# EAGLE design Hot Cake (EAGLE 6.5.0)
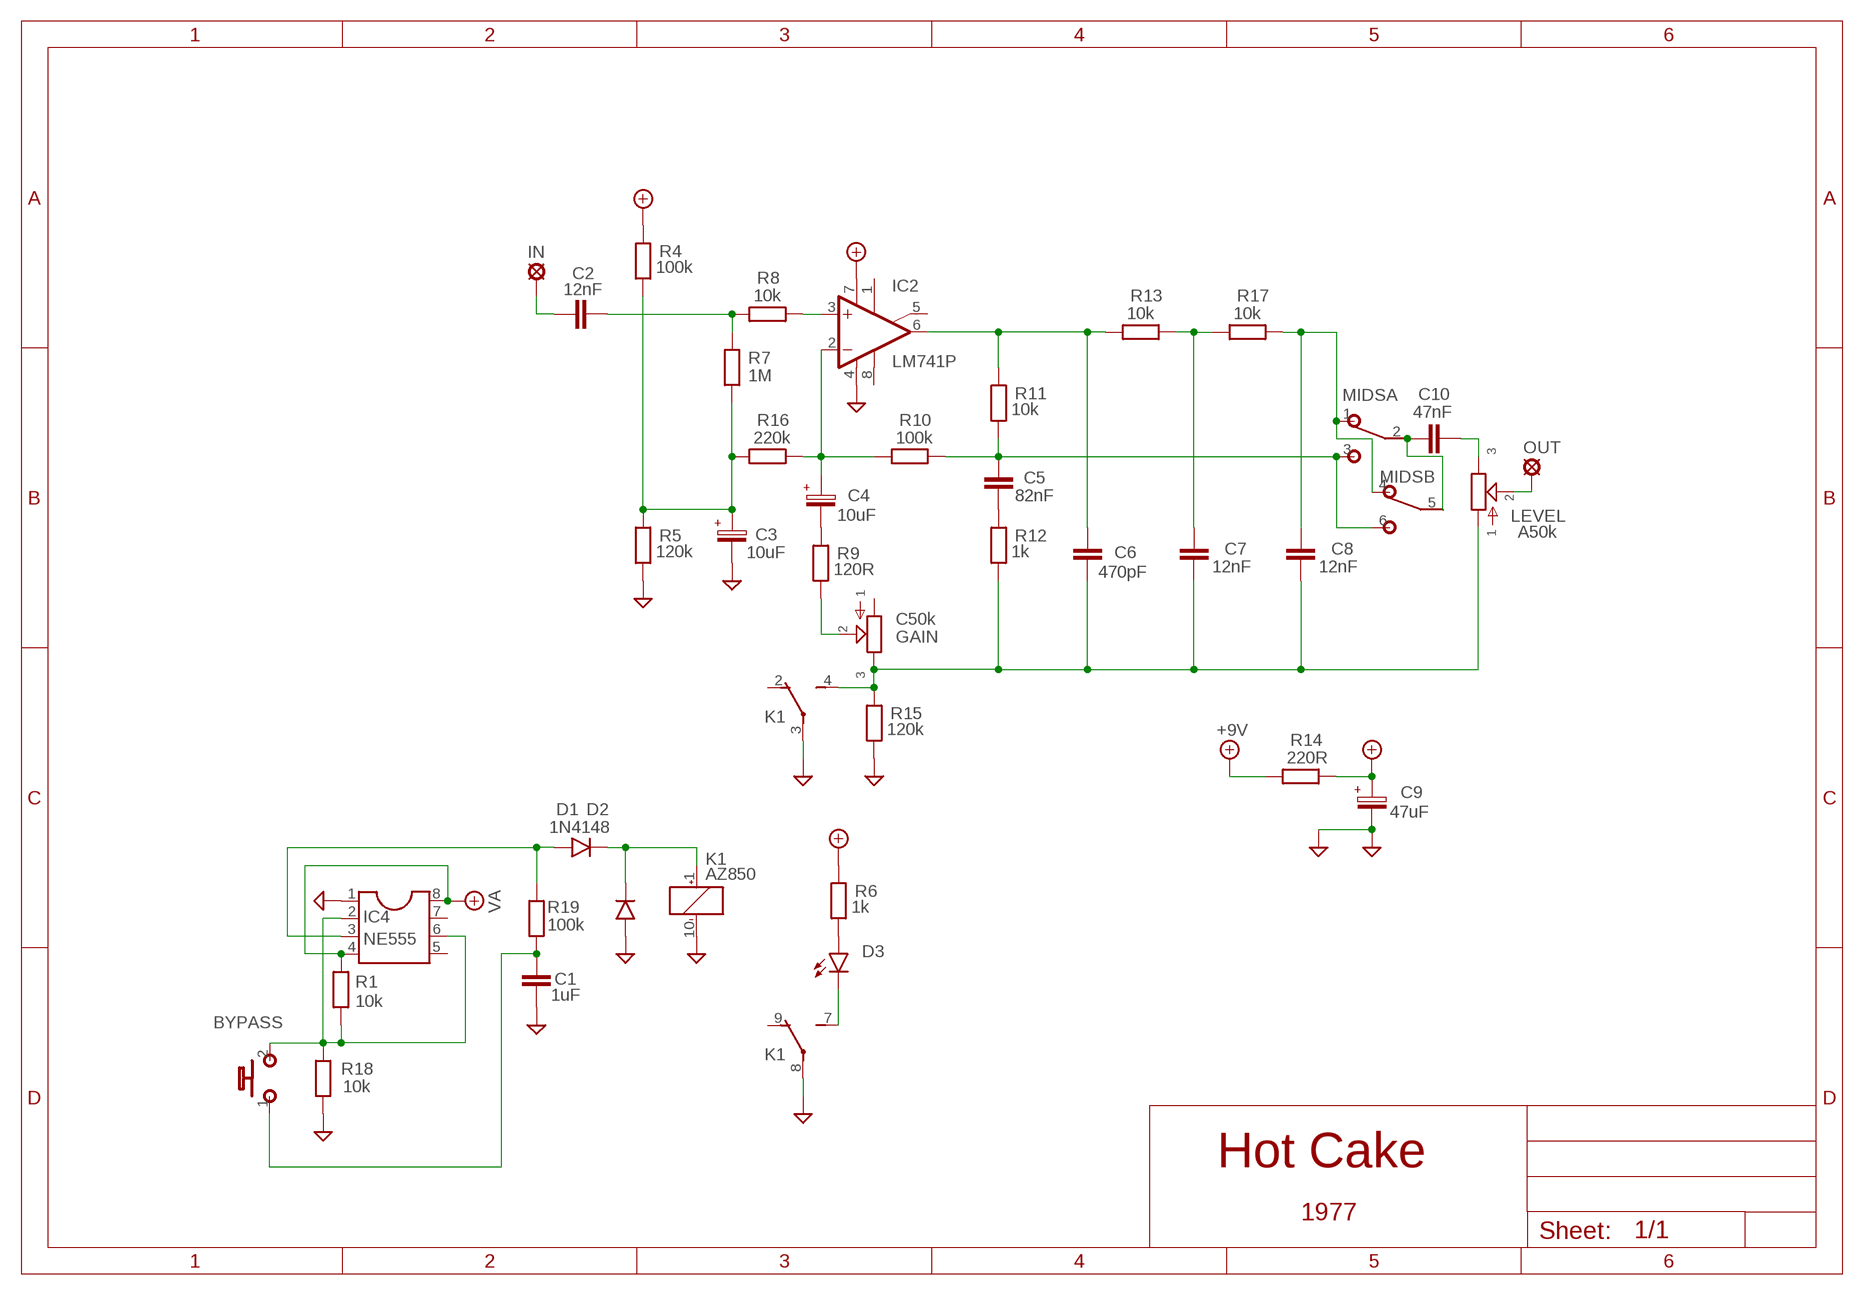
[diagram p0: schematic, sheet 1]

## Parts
+9V  +9V  +9V(T)1  [ROUND]
BYPASS  MOMENTARY  [SPST]
C1  1uF  072X0352  [072X035]
C2  12nF  1NF-15NF  [3,5MM]
C3  10uF  063-EU  [063_025]
C4  10uF  063-EU  [063_025]
C5  82nF  22NF-82NF"  [4,5MM]
C6  470pF  050X030_0251  [050X030_025]
C7  12nF  22NF-82NF"  [4,5MM]
C8  12nF  22NF-82NF"  [4,5MM]
C9  47uF  063-EU  [063_025]
C10  47nF  22NF-82NF"  [4,5MM]
D1  1N4148  1N4148-3  [DO35-3]
D2  1N4005  1N4148-3  [DO35-3]
D3  LED3MM  [LED3MM]
GAIN  C50k  POT-EU16MM  [16MM]
GND  GND(T)1  [ROUND]
GND11  GND(T)1  [ROUND]
IC2  LM741P  [DIL08]
IC4  NE555  DIL8  [DIL08]
IN  MCS10B  [MCS10B]
K1  AZ850  TQ2-5V  [TQ2]
LEVEL  A50k  POT-EU16MM  [16MM]
MIDS  DPDTTHT  [M9040P2]
OUT  MCS10B  [MCS10B]
R1  10k  6MM-EU3  [R0207/3]
R4  100k  6MM-EU1  [R0207/1V]
R5  120k  6MM-EU1  [R0207/1V]
R6  1k  6MM-EU3  [R0207/3]
R7  1M  6MM-EU1  [R0207/1V]
R8  10k  6MM-EU1  [R0207/1V]
R9  120R  6MM-EU3  [R0207/3]
R10  100k  6MM-EU1  [R0207/1V]
R11  10k  6MM-EU1  [R0207/1V]
R12  1k  6MM-EU1  [R0207/1V]
R13  10k  6MM-EU1  [R0207/1V]
R14  220R  6MM-EU3  [R0207/3]
R15  120k  6MM-EU1  [R0207/1V]
R16  220k  6MM-EU1  [R0207/1V]
R17  10k  6MM-EU1  [R0207/1V]
R18  10k  6MM-EU3  [R0207/3]
R19  100k  6MM-EU3  [R0207/3]

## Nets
+9V: +9V.1(+9V) R14.1
GND: C1.2 C3.- C9.- D2.A GND11.1(GND) GND.1(GND) IC2.4(V-) IC4.1 K1.3(1:P) K1.8(2:P) K1.10(_:-) R5.1 R15.1 R18.1
N$1: IC2.3(+IN) R8.2
N$2: C2.2 R7.2 R8.1
N$3: C2.1 IN.MP
N$4: C3.+ R4.1 R5.2 R7.1 R16.1
N$5: C4.+ IC2.2(-IN) R10.1 R16.2
N$6: C5.1 MIDS.3 MIDS.6 R10.2 R11.1
N$7: C6.1 IC2.6(OUT) R11.2 R13.1
N$8: C5.2 R12.2
N$9: C4.- R9.2
N$10: GAIN.2 R9.1
N$12: C8.1 MIDS.1 MIDS.4 R17.2
N$13: C7.1 R13.2 R17.1
N$14: C10.1 MIDS.2 MIDS.5
N$15: LEVEL.2 OUT.MP
N$16: D3.A R6.1
N$17: D3.K(C) K1.7(2:S)
N$18: C10.2 LEVEL.3
N$19: C6.2 C7.2 C8.2 GAIN.3 K1.4(1:S) LEVEL.1 R12.1 R15.2
N$22: BYPASS.2(S) IC4.2 IC4.6 R1.1 R18.2
N$24: D1.A IC4.3 R19.2
N$25: BYPASS.1(P) C1.1 R19.1
N$26: D1.C D2.C K1.1(_:+)
VA: C9.+ IC2.7(V+) IC4.4 IC4.8 R1.2 R4.2 R6.2 R14.2
Unconnected: GAIN.1 IC2.1(ON1) IC2.5(ON2) IC2.8(OPT) IC4.5 IC4.7 K1.2(1:O) K1.9(2:O)

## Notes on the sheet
- 1977

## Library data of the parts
+9V = Virransyöttö:+9V(T): +9V Voltage Supply
BYPASS = Kytkimet:MOMENTARY
C1 = Wima MKS:072X035: 0.15 - 1.0uF;
C2 = Mylar Kondensaattorit:1NF-15NF: 1nF-15nF
C3 C4 C9 = Elektrolyytit:063-EU
C5 C7 C8 C10 = Mylar Kondensaattorit:22NF-82NF: 22nF-82nF
C6 = Keraamiset kondensaattorit:050X030_025: 47 - 120pF
D1 D2 = Diodit:1N4148: Fast Switching Diode
D3 = Diodit:LED
GAIN LEVEL = potentiometers:POT-EU
GND GND11 = Virransyöttö:GND(T): Ground
IC2 = Operaatiovahvistimet:*741: OP AMP
IC4 = ic-package:DIL8: Dual In Line / Socket
IN OUT = Padit:MCS10B: SOLDER PAD
K1 = relay:TQ2?*: LOW PROFILE 2 FORM C RELAY NAiS Source: http://www.mew-europe.com/.. en_ds_61020_0001.pdf Source: http://www.mew-europe.com/.. en_ds_61020_0004.pdf; MF: AROMAT/ MATSUSHITA; MPN: TQ2-5V; OC_FARNELL: 1175716; OC_NEWARK: 64K3200
MIDS = Kytkimet:DPDT
R1 R4-R19 = gm-resistors:6MM-EU: 6mm Resistors (European schematic symbol)

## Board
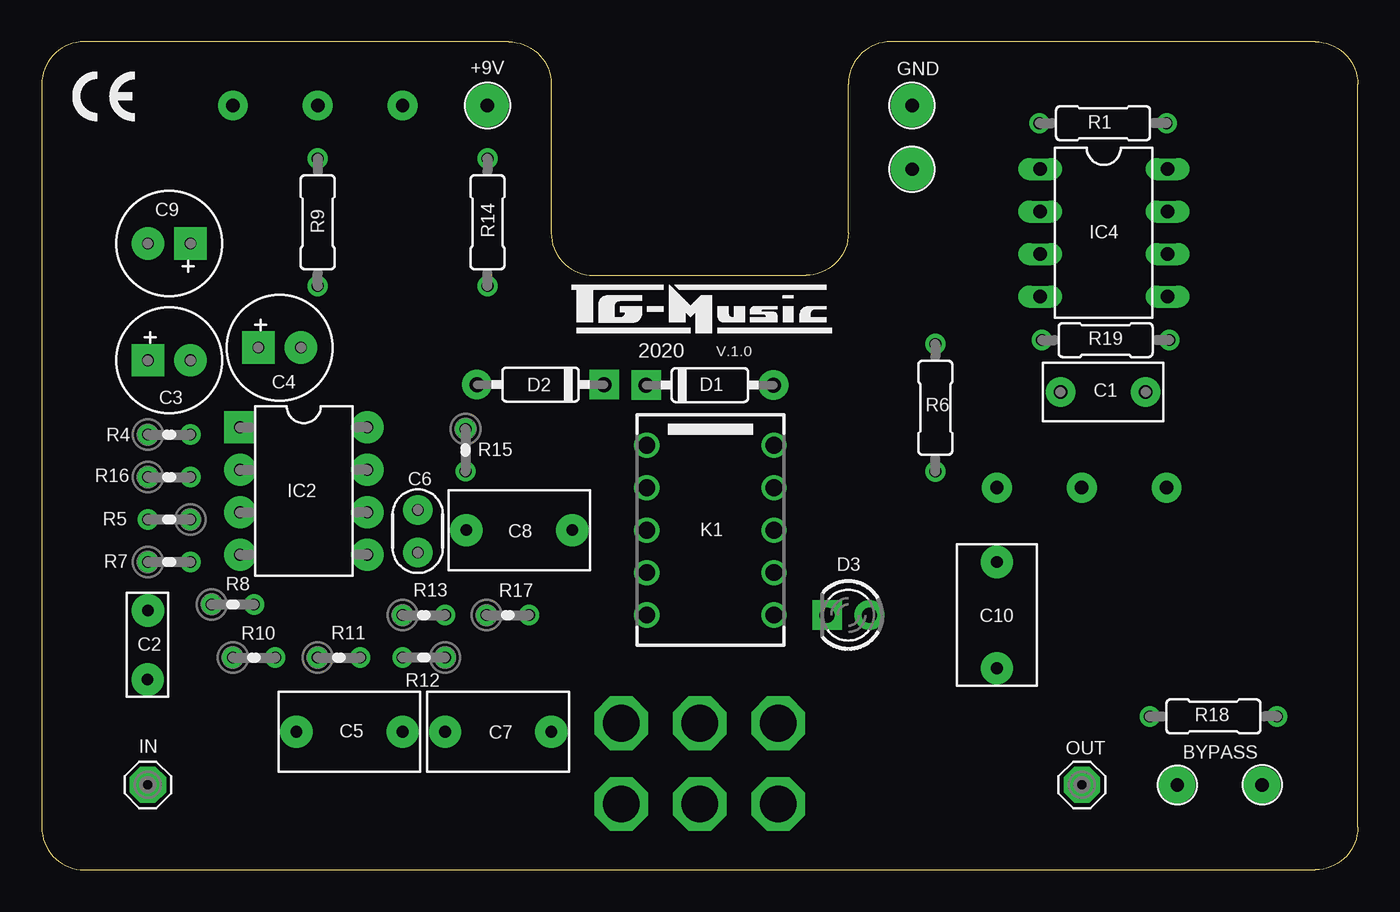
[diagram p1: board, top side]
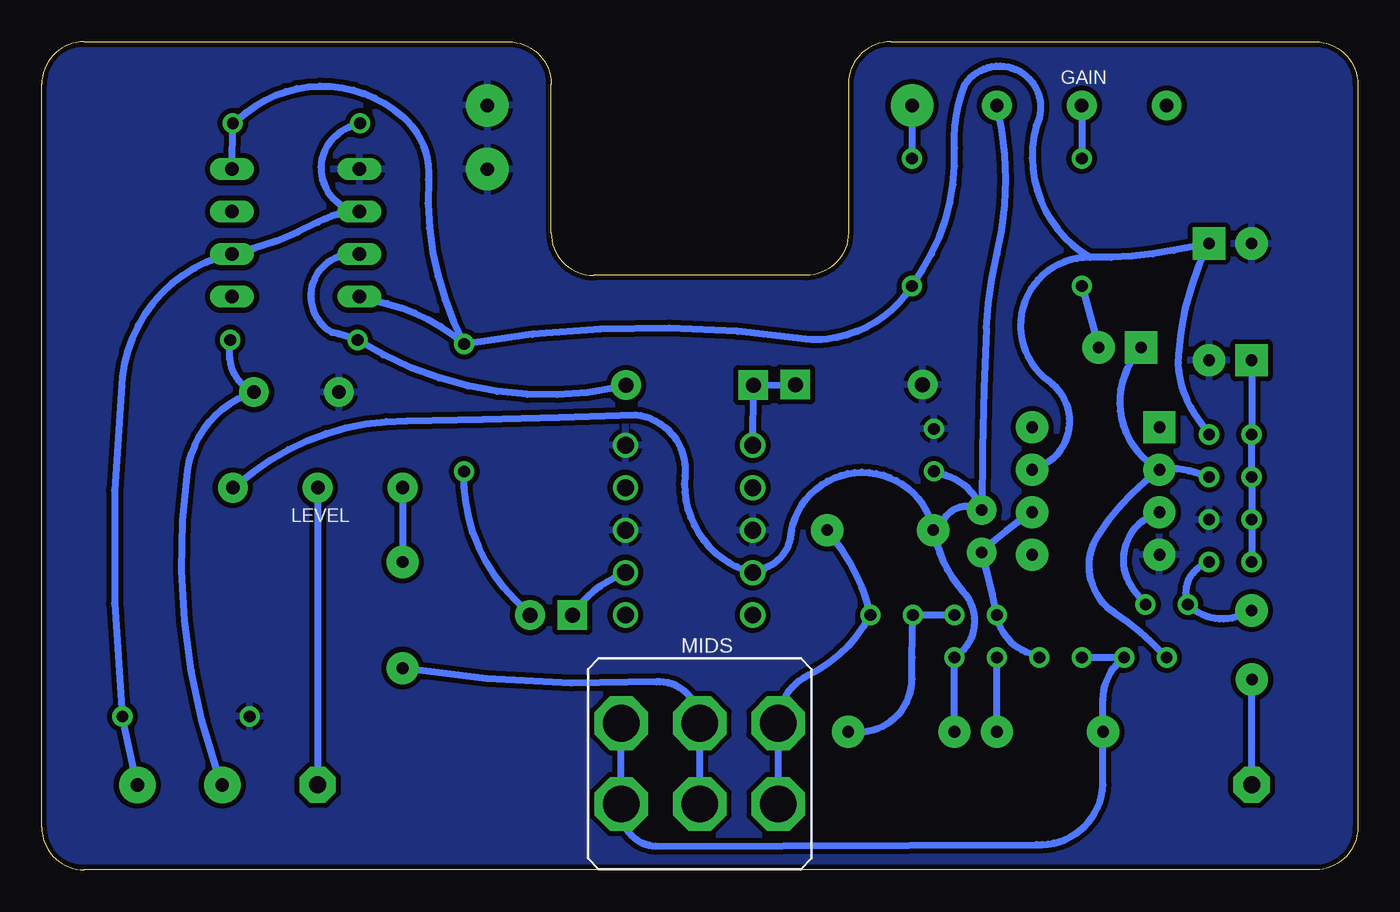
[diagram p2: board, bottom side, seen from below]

Size 78.74 x 49.53 mm. Coordinates in mm from the lower left corner, seen from the top.
Outline: 7.62,49.53 3.81,49.53
Outline: 78.74,2.54 78.74,46.99 arc90 76.2,49.53 50.8,49.53 arc90 48.26,46.99 48.26,38.1 arc-90 45.72,35.56 33.02,35.56 arc-90 30.48,38.1 30.48,46.99 arc90 27.94,49.53 2.54,49.53 arc90 0,46.99 0,2.54 arc90 2.54,0 76.2,0 arc90 78.74,2.54
Copper layers (1*16): Top 0.035mm / dielectric 1.5mm / Bottom 0.035mm
Design rules "ITEADstudio": minimum track width 10mil, minimum drill 12mil, track to track 12mil, track to pad 12mil, pad to pad 12mil, via to via 12mil, smd to smd 0mil, copper to edge 12mil, drill to drill 12mil, minimum pad ring 10mil, minimum via ring 6mil, stop-mask expansion 4mil, vias tented up to drill 100mil, thermal gap 10mil

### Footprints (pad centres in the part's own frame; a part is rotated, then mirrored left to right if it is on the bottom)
ROUND = drill 0.8 pad 2.54: 1 0,0
SPST = drill 0.8 pad 2.184: 1 -2.54,0; 2 2.54,0
072X035 = drill 0.8 pad 1.778: 1 -2.54,0; 2 2.54,0
3,5MM = drill 0.7 pad 1.93: 1 -1.905,0; 2 2.221,-0.016
063_025 = drill 0.7 pad 1.93 square: + -1.27,0 | drill 0.7 pad 1.93: - 1.27,0
4,5MM = drill 0.7 pad 1.93: 1 -3.175,0; 2 3.175,0
050X030_025 = drill 0.7 pad 1.778: 1 -1.27,0; 2 1.27,0
DO35-3 = drill 0.9 pad 1.778: A 3.81,0 | drill 0.9 pad 1.778 square: C -3.81,0
LED3MM = drill 0.9 pad 1.778: A -1.27,0 | drill 0.9 pad 1.778 square: K 1.27,0
16MM = drill 0.8 pad 1.778: 1 5.08,0; 2 0,0; 3 -5.08,0
DIL08 = drill 0.7 pad 1.93 square: 1 -3.81,-3.81 | drill 0.7 pad 1.93: 2 -1.27,-3.81; 3 1.27,-3.81; 4 3.81,-3.81; 5 3.81,3.81; 6 1.27,3.81; 7 -1.27,3.81; 8 -3.81,3.81
DIL08' = drill 0.813 long: 1 -3.81,-3.81; 2 -1.27,-3.81; 3 1.27,-3.81; 4 3.81,-3.81; 5 3.81,3.81; 6 1.27,3.81; 7 -1.27,3.81; 8 -3.81,3.81
MCS10B = drill 1.016 pad 2.159 octagon: MP 0,0
TQ2 = drill 1: 1 -5.08,-3.81; 2 -2.54,-3.81; 3 0,-3.81; 4 2.54,-3.81; 5 5.08,-3.81; 6 5.08,3.81; 7 2.54,3.81; 8 0,3.81; 9 -2.54,3.81; 10 -5.08,3.81
M9040P2 = drill 2.2 octagon: 1 -2.413,4.699; 2 -2.413,0; 3 -2.413,-4.699; 4 2.413,4.699; 5 2.413,0; 6 2.413,-4.699
R0207/3 = drill 0.7: 1 -3.81,0; 2 3.81,0
R0207/1V = drill 0.7: 1 -1.27,0; 2 1.27,0

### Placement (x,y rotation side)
+9V  26.67,45.72 0 top
BYPASS  70.48,5.08 0 top
C1  63.5,28.57 180 top
C2  6.33,13.3 90 top
C3  7.62,30.48 0 top
C4  14.23,31.24 0 top
C5  18.41,8.26 0 top
C6  22.5,20.26 90 top
C7  27.3,8.26 180 top
C8  28.57,20.32 180 top
C9  7.62,37.47 180 top
C10  57.15,15.24 90 top
D1  39.97,29 0 top
D2  29.84,29.03 180 top
D3  48.26,15.24 180 top
GAIN  16.51,45.72 0 bottom
GND  52.07,45.72 0 top
GND11  52.07,41.91 0 top
IC2  15.67,22.66 270 top
IC4  NE555  [DIL08']  63.54,38.1 270 top
IN  6.35,5.08 0 top
K1  40.01,20.32 270 top
LEVEL  62.23,22.86 180 bottom
MIDS  39.37,6.35 270 bottom
OUT  62.23,5.08 0 top
R1  63.5,44.66 0 top
R4  7.62,26.04 0 top
R5  7.62,20.95 180 top
R6  53.47,27.64 90 top
R7  7.62,18.41 0 top
R8  11.43,15.88 0 top
R9  16.51,38.73 270 top
R10  12.7,12.7 0 top
R11  17.78,12.7 0 top
R12  22.86,12.7 180 top
R13  22.86,15.24 0 top
R14  26.67,38.73 270 top
R15  25.35,25.11 270 top
R16  7.62,23.5 0 top
R17  27.88,15.24 0 top
R18  70.11,9.18 0 top
R19  63.66,31.69 180 top

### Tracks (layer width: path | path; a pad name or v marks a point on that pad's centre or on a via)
+9V
  Bottom 0.406: +9V.1 R14.1
GND
  pour Bottom: 0,2.54 0,46.99 arc-90 2.54,49.53 27.94,49.53 arc-90 30.48,46.99 30.48,38.1 arc90 33.02,35.56 45.72,35.56 arc90 48.26,38.1 48.26,46.99 arc-90 50.8,49.53 76.2,49.53 arc-90 78.74,46.99 78.74,2.54 arc-90 76.2,0 2.54,0 arc-90
N$1
  Bottom 0.406: R8.2 13.35,16.68 arc113 IC2.3
N$2
  Bottom 0.406: C2.2 6.99,15.24 arc70 R8.1 arc86 9.23,18.25 R7.2
N$3
  Bottom 0.406: IN.MP C2.1
N$4
  Bottom 0.406: C3.+ R4.1 R16.1 R5.2 R7.1
N$5
  Bottom 0.406: R16.2 9.77,23.78 arc-27 IC2.2 | C4.+ 13.31,30.76 arc-98 IC2.2 | R10.1 12.36,13.62 arc-12 14.52,15.35 arc90 15.52,20.02 arc20 IC2.2
N$6
  Bottom 0.406: R11.1 R10.2 arc-53 15.24,10.16 C5.1 15.24,5.08 arc90 19.23,1.51 42,1.42 arc97 MIDS.6 MIDS.3
N$7
  Bottom 0.406: R11.2 19.86,13.04 arc58 R13.1 arc-5 C6.1 arc10 20.26,20.85 IC2.6
N$8
  Bottom 0.406: C5.2 R12.2
N$9
  Bottom 0.406: R9.2 C4.-
N$10
  Bottom 0.406: GAIN.2 R9.1
N$12
  Bottom 0.406: C8.1 31.36,19.81 arc24 R17.2 arc35 32.88,11.64 arc-64 MIDS.1 MIDS.4
N$13
  Bottom 0.406: R13.2 R17.1 arc-2 26.67,11.43 arc90 29.84,8.26 C7.1
N$14
  Bottom 0.406: MIDS.5 MIDS.2 arc-93 41.98,11.25 arc12 C10.1
N$15
  Bottom 0.406: LEVEL.2 OUT.MP
N$16
  Bottom 0.406: D3.A 50.44,16.18 arc48 R6.1
N$17
  Bottom 0.406: K1.7 44.5,17.44 arc-31 D3.K
N$18
  Bottom 0.406: LEVEL.3 C10.2
N$19
  Bottom 0.406: C8.2 24.77,20.95 arc90 C6.2 | C7.2 R12.1 arc-100 23.61,16.64 arc27 25.17,19.49 C8.2 | C6.2 arc2 22.23,32.38 arc11 21.59,36.83 arc-28 GAIN.3 | C8.2 arc-158 33.88,20.26 arc67 35.46,18.06 arc71 K1.4 arc81 40.26,23.6 arc-89 43.22,27.22 arc1 56.91,26.85 arc-38 66.06,23.81 LEVEL.1 | R15.2 24.66,23.61 arc52 C6.2
N$22
  Bottom 0.406: R1.1 60.35,44.41 arc-152 IC4.2 arc-28 62.23,38.73 arc16 IC4.6 arc-72 73.92,29.46 arc-12 R18.2 BYPASS.2
N$24
  Bottom 0.406: D1.A 44.34,28.83 arc44 R19.2 arc-12 61.39,32.15 arc157 IC4.3
N$25
  Bottom 0.406: BYPASS.1 68.3,6.1 arc27 70.02,23.88 arc65 C1.1 arc70 67.51,31.02 R19.1
N$26
  Bottom 0.406: D2.C D1.C K1.1
VA
  Bottom 0.406: 16.01,36.63 arc-12 11.03,37.05 C9.+ arc-23 10.71,30.8 arc-39 9.73,27.25 R4.2 | 16.01,36.63 arc-92 20.18,32.49 arc-53 18.49,29.24 arc129 IC2.7 | R6.2 arc31 55.6,41.31 arc-52 57.12,45.04 arc-80 66.52,45.29 R1.2 IC4.8 | IC4.4 58.92,34.07 arc30 R6.2 | R6.2 arc18 33.02,31.75 arc-13 31.75,31.75 arc-51 R14.2 26.05,35.9 arc-36 24.13,43.18 arc25 23.5,46.97 arc173 19.23,44.52 arc-75 16.01,36.63

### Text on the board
tNames: 2020 | V.1.0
